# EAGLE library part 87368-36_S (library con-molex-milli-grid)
RECEPTACAL
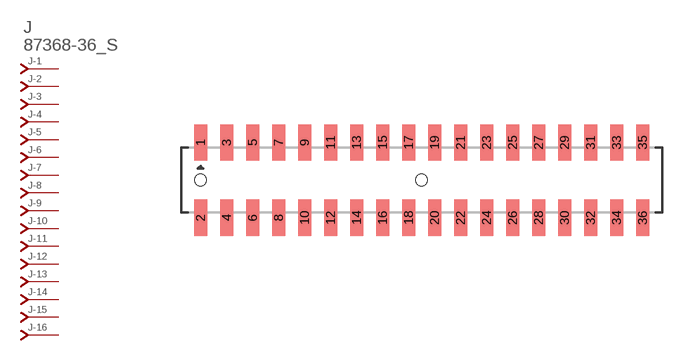
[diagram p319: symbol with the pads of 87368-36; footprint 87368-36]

Designator prefix J; gates -1=J-NV -2=J-N -3=J-N -4=J-N -5=J-N -6=J-N -7=J-N -8=J-N -9=J-N -10=J-N -11=J-N -12=J-N -13=J-N -14=J-N -15=J-N -16=J-N -17=J-N -18=J-N -19=J-N -20=J-N -21=J-N -22=J-N -23=J-N -24=J-N -25=J-N -26=J-N -27=J-N -28=J-N -29=J-N -30=J-N -31=J-N -32=J-N -33=J-N -34=J-N -35=J-N -36=J-N

## 87368-36_S  [87368-36]
1  -1:J  pas
2  -2:J  pas
3  -3:J  pas
4  -4:J  pas
5  -5:J  pas
6  -6:J  pas
7  -7:J  pas
8  -8:J  pas
9  -9:J  pas
10  -10:J  pas
11  -11:J  pas
12  -12:J  pas
13  -13:J  pas
14  -14:J  pas
15  -15:J  pas
16  -16:J  pas
17  -17:J  pas
18  -18:J  pas
19  -19:J  pas
20  -20:J  pas
21  -21:J  pas
22  -22:J  pas
23  -23:J  pas
24  -24:J  pas
25  -25:J  pas
26  -26:J  pas
27  -27:J  pas
28  -28:J  pas
29  -29:J  pas
30  -30:J  pas
31  -31:J  pas
32  -32:J  pas
33  -33:J  pas
34  -34:J  pas
35  -35:J  pas
36  -36:J  pas

## Footprint 87368-36 (pad centres in mm)
RECEPTACAL SMD Dual Row, Side Entry
smd 1 x 2.8: 1 -17,2.9; 2 -17,-2.9; 3 -15,2.9; 4 -15,-2.9; 5 -13,2.9; 6 -13,-2.9; 7 -11,2.9; 8 -11,-2.9; 9 -9,2.9; 10 -9,-2.9; 11 -7,2.9; 12 -7,-2.9; 13 -5,2.9; 14 -5,-2.9; 15 -3,2.9; 16 -3,-2.9; 17 -1,2.9; 18 -1,-2.9; 19 1,2.9; 20 1,-2.9; 21 3,2.9; 22 3,-2.9; 23 5,2.9; 24 5,-2.9; 25 7,2.9; 26 7,-2.9; 27 9,2.9; 28 9,-2.9; 29 11,2.9; 30 11,-2.9; 31 13,2.9; 32 13,-2.9; 33 15,2.9; 34 15,-2.9; 35 17,2.9; 36 17,-2.9
hole 0.914 at -17,0
hole 0.914 at 0,0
